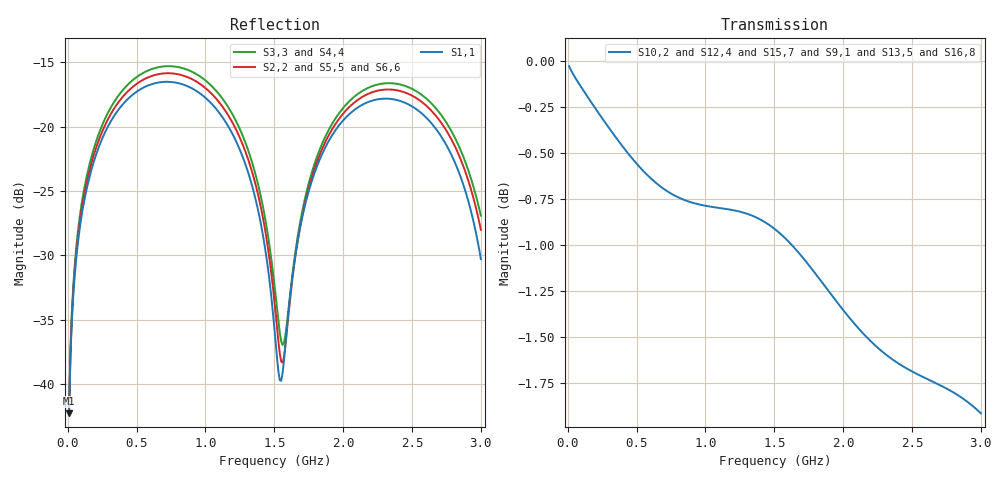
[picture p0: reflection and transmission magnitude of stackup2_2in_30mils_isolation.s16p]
! Touchstone file from project
# GHZ S RI R 50.000000
! Modal data exported
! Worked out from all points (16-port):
!   300 points, 10 MHz to 3 GHz, reference 50 ohm
!   strongest paths, dB at 10 MHz, 760 MHz, 1.51 GHz, 2.26 GHz, 3 GHz:
!     S10,2: 0.0, -0.7, -0.9, -1.6, -1.9
!     S12,4: 0.0, -0.7, -0.9, -1.6, -1.9
!     S15,7: 0.0, -0.7, -0.9, -1.6, -1.9
!     S9,1: 0.0, -0.7, -0.9, -1.6, -1.9
!     S13,5: 0.0, -0.7, -0.9, -1.6, -1.9
!     S16,8: 0.0, -0.7, -0.9, -1.6, -1.9
!   lowest |S11| = -42.3 dB at 10 MHz (marker M1), VSWR 1.02, Z = 50.3 + j0.705 ohm
!   |S11| at or under -10 dB: start of sweep to end of sweep
